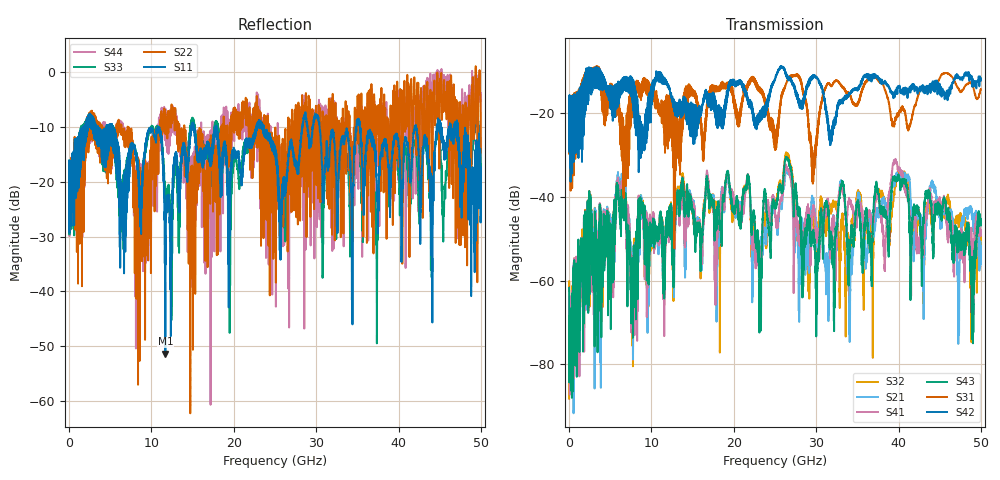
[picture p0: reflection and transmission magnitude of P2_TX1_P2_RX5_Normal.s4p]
!Keysight Technologies,N5225B,MY57041031,A.13.20.10
!Date: Friday, May 31, 2019 11:34:05
!Correction: S11(Full 4 Port(1,2,3,4))
!S12(Full 4 Port(1,2,3,4))
!S13(Full 4 Port(1,2,3,4))
!S14(Full 4 Port(1,2,3,4))
!S21(Full 4 Port(1,2,3,4))
!S22(Full 4 Port(1,2,3,4))
!S23(Full 4 Port(1,2,3,4))
!S24(Full 4 Port(1,2,3,4))
!S31(Full 4 Port(1,2,3,4))
!S32(Full 4 Port(1,2,3,4))
!S33(Full 4 Port(1,2,3,4))
!S34(Full 4 Port(1,2,3,4))
!S41(Full 4 Port(1,2,3,4))
!S42(Full 4 Port(1,2,3,4))
!S43(Full 4 Port(1,2,3,4))
!S44(Full 4 Port(1,2,3,4))
!S4P File: Measurements: <S11,S12,S13,S14>,
!<S21,S22,S23,S24>,
!<S31,S32,S33,S34>,
!<S41,S42,S43,S44>:
# Hz S  dB  R 50.0
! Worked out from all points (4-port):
!   5000 points, 10 MHz to 50 GHz, reference 50 ohm
!   strongest paths, dB at 10 MHz, 12.51 GHz, 25.01 GHz, 37.51 GHz, 50 GHz:
!     S42: -19.5, -16.7, -11.8, -11.1, -11.6
!     S31: -19.5, -17.3, -28.8, -12.1, -14.2
!     S43: -61.7, -45.2, -41.9, -38.0, -46.7
!     S41: -62.6, -44.6, -43.1, -39.2, -48.0
!     S21: -63.5, -44.3, -43.9, -43.2, -51.7
!     S32: -88.2, -45.3, -42.6, -39.1, -51.8
!   lowest |S11| = -51.4 dB at 11.69 GHz (marker M1), VSWR 1.01, Z = 49.8 - j0.169 ohm
!   |S11| at or under -10 dB: 5.36 GHz to 10.81 GHz (5.449 GHz wide, 67.4 % of centre); 17.89 GHz to 22.7 GHz (4.805 GHz wide, 23.7 % of centre); 35.31 GHz to 41.95 GHz (6.643 GHz wide, 17.2 % of centre)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
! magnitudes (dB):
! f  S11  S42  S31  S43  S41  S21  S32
! 10 MHz  -19.6  -19.5  -19.5  -61.7  -62.6  -63.5  -88.2
! 5.97 GHz  -21.0  -12.8  -18.2  -38.0  -36.9  -36.0  -37.1
! 11.69 GHz  -51.4  -13.0  -23.0  -49.5  -51.2  -50.5  -49.9
! 23.19 GHz  -9.0  -19.4  -14.2  -59.7  -56.8  -52.2  -54.4
! 26.46 GHz  -19.9  -11.0  -12.3  -30.6  -33.0  -33.6  -29.5
! 30.1 GHz  -8.3  -11.5  -25.3  -56.6  -49.9  -49.0  -53.1
! 50 GHz  -17.4  -11.6  -14.2  -46.7  -48.0  -51.7  -51.8
